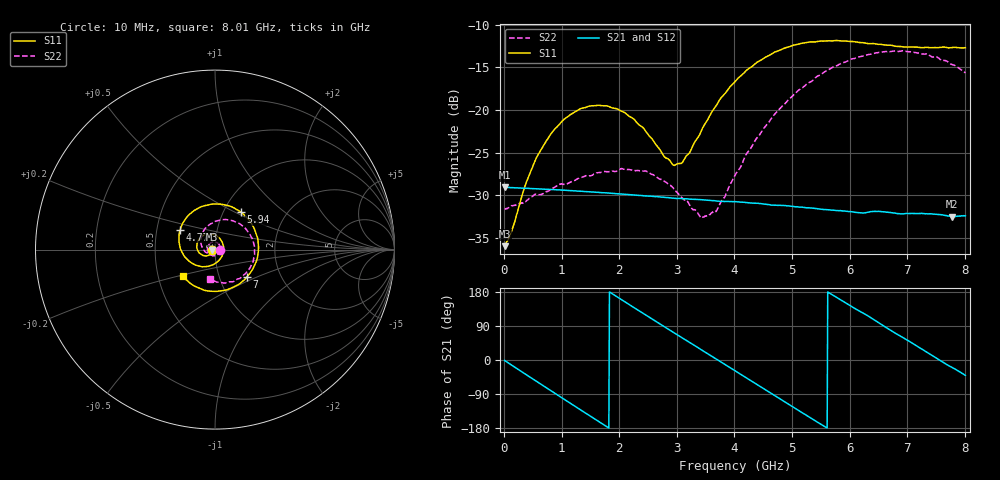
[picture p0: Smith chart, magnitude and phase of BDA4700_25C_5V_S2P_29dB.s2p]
!Agilent Technologies,E5071B,MY42404982,A.09.10
!Date: Mon Oct 20 13:41:10 2025
!Data & Calibration Information:
!Freq	S11:SOLT2(ON)	S21:SOLT2(ON)	S12:SOLT2(ON)	S22:SOLT2(ON)
# Hz S RI R 50
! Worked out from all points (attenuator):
!   801 points, 10 MHz to 8.01 GHz, reference 50 ohm
!   highest |S21| = -29.07 dB at 10 MHz (marker M1); lowest = -32.5 dB at 7.77 GHz (marker M2)
!   lowest |S11| = -36.0 dB at 10 MHz (marker M3), VSWR 1.03, Z = 48.4 - j0.118 ohm
!   |S11| at or under -10 dB: start of sweep to end of sweep
!   |S22| runs from -32.7 to -13.0 dB; largest |S21 - S12| = 0.0003
!   S11 on the Smith chart (normalised r, x): 10 MHz: 0.97, -0.00; 4.77 GHz: 0.66, +0.15; 5.94 GHz: 1.20, +0.54; 7 GHz: 1.35, -0.44; 8.01 GHz: 0.67, -0.21
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1e7  -0.0158 -0.00121  0.0352 -0.000758  0.0352 -0.000758  0.0262 -0.000807
1.2e8  -0.0168 -0.00858  0.0342 -0.00745  0.0342 -0.00747  0.0266 -0.00578
6e8  -0.0431 -0.0346  0.0172 -0.0298  0.0172 -0.0298  0.0128 -0.0291
1e9  -0.082 -0.0236  -0.00549 -0.0334  -0.00549 -0.0334  -0.0146 -0.0338
1.35e9  -0.1018 0.0122  -0.023 -0.0241  -0.023 -0.0241  -0.036 -0.0178
2.07e9  -0.0451 0.0863  -0.0294 0.0128  -0.0293 0.0129  -0.0305 0.033
2.68e9  0.0374 0.0471  -0.00415 0.0306  -0.00414 0.0306  0.0127 0.0375
2.93e9  0.0474 0.00549  0.00842 0.0291  0.00846 0.0291  0.0246 0.0248
3.06e9  0.045 -0.0179  0.0144 0.0266  0.0143 0.0266  0.0274 0.0149
3.44e9  0.000657 -0.0774  0.0268 0.0128  0.0268 0.0128  0.0187 -0.0139
3.69e9  -0.0504 -0.0943  0.0292 0.001  0.0292 0.000898  0.0007 -0.0256
4.01e9  -0.1244 -0.0777  0.0254 -0.0137  0.0255 -0.0137  -0.0321 -0.0258
4.41e9  -0.1924 0.00402  0.0113 -0.026  0.0113 -0.026  -0.0693 0.00733
4.77e9  -0.1935 0.1111  -0.00497 -0.0271  -0.00485 -0.0271  -0.0787 0.0619
5.35e9  -0.0629 0.2434  -0.0241 -0.0111  -0.0241 -0.0111  -0.0154 0.1473
5.94e9  0.1425 0.2105  -0.0219 0.0128  -0.022 0.0128  0.1166 0.1529
6.37e9  0.2327 0.0785  -0.00924 0.0235  -0.00924 0.0235  0.197 0.0803
6.68e9  0.2368 -0.0422  0.00379 0.0248  0.00381 0.0248  0.22 0.000603
7e9  0.1778 -0.1531  0.015 0.0196  0.0151 0.0195  0.2032 -0.0851
7.37e9  0.0522 -0.2269  0.0233 0.00753  0.0234 0.0075  0.1376 -0.1614
7.77e9  -0.107 -0.207  0.0223 -0.00771  0.0224 -0.00773  0.029 -0.1833
8.01e9  -0.1792 -0.1478  0.0181 -0.0156  0.0182 -0.0156  -0.0302 -0.1626
